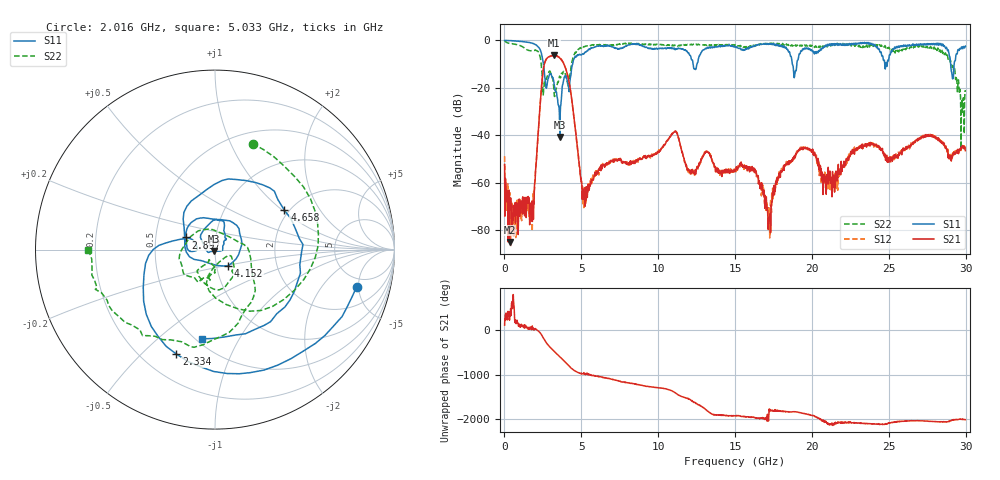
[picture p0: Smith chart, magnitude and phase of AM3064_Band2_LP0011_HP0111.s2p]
# Hz S DB R 50.0
!freq dBS11 angS11 dBS21 angS21 dBS12 angS12 dBS22 angS22
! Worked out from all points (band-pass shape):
!   1600 points, 10 MHz to 29.98 GHz, reference 50 ohm
!   highest |S21| = -6.28 dB at 3.234 GHz (marker M1); lowest = -85.1 dB at 328.6 MHz (marker M2)
!   |S21| within 3 dB of the highest: 2.631 GHz to 3.816 GHz (1.185 GHz wide, 36.8 % of centre)
!   lowest |S11| = -40.7 dB at 3.609 GHz (marker M3), VSWR 1.02, Z = 49.5 - j0.779 ohm
!   |S11| at or under -10 dB: 2.539 GHz to 4.434 GHz (1.895 GHz wide, 54.4 % of centre); 12.27 GHz to 12.52 GHz (255.8 MHz wide, 2.06 % of centre); 18.73 GHz to 19.02 GHz (294.9 MHz wide, 1.56 % of centre)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
!   |S22| runs from -45.8 to -0.2 dB; largest |S21 - S12| = 0.019
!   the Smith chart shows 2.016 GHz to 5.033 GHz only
!   S11 on the Smith chart (normalised r, x): 2.016 GHz: 3.81, -4.74; 2.334 GHz: 0.34, -0.64; 2.897 GHz: 0.72, +0.10; 4.152 GHz: 1.14, -0.21; 4.658 GHz: 1.89, +1.03; 5.033 GHz: 0.53, -0.71
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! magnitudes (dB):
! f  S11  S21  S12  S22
! 10 MHz  -0.1  -52.4  -48.9  -0.2
! 328.6 MHz  -0.1  -85.1  -72.9  -1.3
! 1.734 GHz  -1.1  -72.0  -71.8  -4.4
! 2.016 GHz  -1.8  -55.6  -55.6  -4.1
! 2.334 GHz  -4.1  -26.1  -25.9  -7.4
! 2.897 GHz  -15.1  -6.9  -6.9  -13.2
! 3.234 GHz  -18.6  -6.3  -6.5  -22.5
! 3.609 GHz  -40.7  -7.5  -7.5  -15.4
! 4.152 GHz  -18.7  -16.1  -16.0  -19.9
! 4.658 GHz  -7.0  -40.2  -40.0  -5.0
! 5.015 GHz  -6.1  -59.4  -60.9  -3.2
! 5.033 GHz  -6.0  -60.2  -62.5  -3.0
! 10 GHz  -3.5  -46.9  -47.5  -1.8
! 15 GHz  -2.6  -54.6  -55.6  -1.8
! 16.26 GHz  -2.4  -55.8  -55.3  -2.3
! 17.2 GHz  -1.6  -76.0  -70.6  -1.5
! 18.15 GHz  -2.8  -53.0  -53.0  -2.0
! 19.99 GHz  -4.2  -46.3  -46.6  -2.1
! 21.3 GHz  -1.9  -66.0  -60.0  -1.5
! 25 GHz  -8.0  -51.1  -50.5  -2.9
! 28.56 GHz  -2.1  -44.1  -43.3  -4.7
! 29.98 GHz  -2.4  -46.5  -45.9  -21.6
